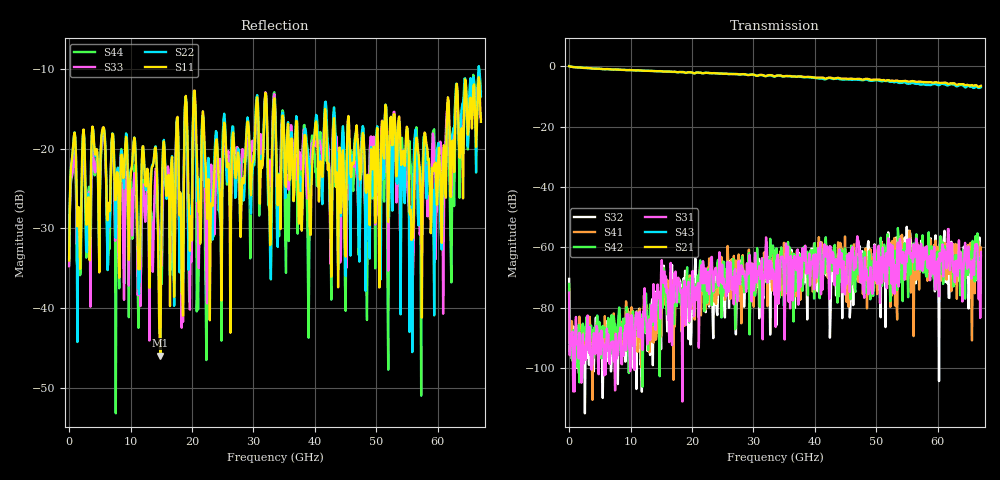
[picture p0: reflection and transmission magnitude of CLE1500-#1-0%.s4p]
!Keysight Technologies,N5247B,US50470101,A.16.20.02
!Date: Thursday, March 13, 2025 10:05:33
!Correction: S11(C  4-Port  )
!S12(C  4-Port  )
!S13(C  4-Port  )
!S14(C  4-Port  )
!S21(C  4-Port  )
!S22(C  4-Port  )
!S23(C  4-Port  )
!S24(C  4-Port  )
!S31(C  4-Port  )
!S32(C  4-Port  )
!S33(C  4-Port  )
!S34(C  4-Port  )
!S41(C  4-Port  )
!S42(C  4-Port  )
!S43(C  4-Port  )
!S44(C  4-Port  )
!S4P File: Measurements: <S11,S12,S13,S14>,
!<S21,S22,S23,S24>,
!<S31,S32,S33,S34>,
!<S41,S42,S43,S44>:
# Hz S  dB  R 50
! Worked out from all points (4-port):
!   601 points, 10 MHz to 67 GHz, reference 50 ohm
!   strongest paths, dB at 10 MHz, 16.76 GHz, 33.51 GHz, 50.25 GHz, 67 GHz:
!     S21: 0.0, -1.9, -3.3, -4.4, -6.5
!     S43: 0.0, -1.9, -3.4, -4.7, -6.9
!     S31: -75.0, -92.4, -69.0, -65.6, -61.5
!     S42: -72.1, -74.4, -64.9, -63.0, -70.9
!     S41: -73.9, -70.8, -74.0, -61.0, -60.0
!     S32: -70.4, -65.8, -73.9, -73.3, -62.8
!   lowest |S11| = -45.9 dB at 14.86 GHz (marker M1), VSWR 1.01, Z = 50.5 + j0.0185 ohm
!   |S11| at or under -10 dB: start of sweep to end of sweep
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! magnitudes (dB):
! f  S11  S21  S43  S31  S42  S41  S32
! 10 MHz  -34.0  0.0  0.0  -75.0  -72.1  -73.9  -70.4
! 13.85 GHz  -20.9  -1.6  -1.6  -81.2  -77.7  -78.5  -79.3
! 14.86 GHz  -45.9  -1.6  -1.7  -83.6  -78.1  -80.4  -84.0
! 19.66 GHz  -32.8  -2.0  -2.0  -81.7  -71.1  -69.3  -82.5
! 20.44 GHz  -12.7  -2.4  -2.3  -78.1  -72.2  -83.9  -69.3
! 55.61 GHz  -27.7  -5.0  -5.6  -63.5  -61.7  -75.0  -57.9
! 67 GHz  -16.7  -6.5  -6.9  -61.5  -70.9  -60.0  -62.8
